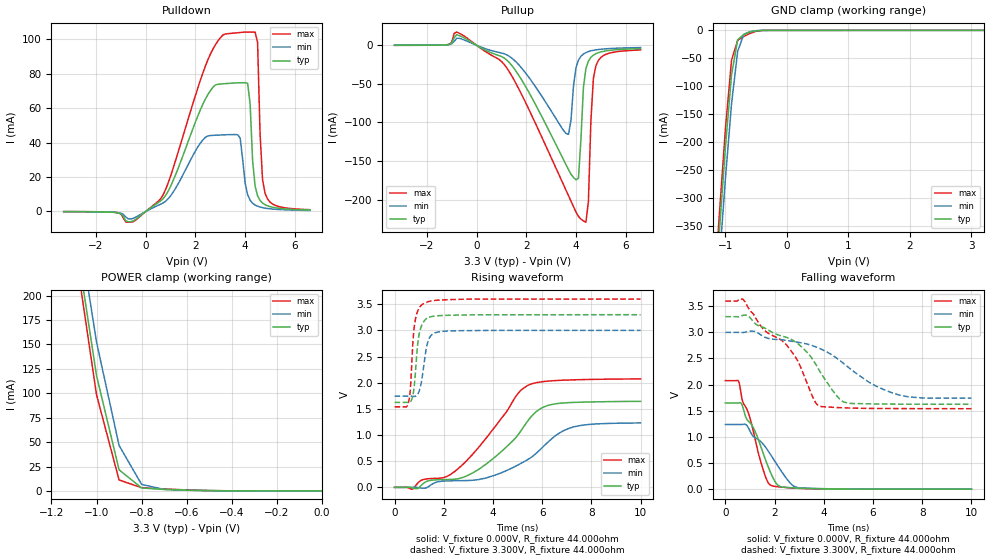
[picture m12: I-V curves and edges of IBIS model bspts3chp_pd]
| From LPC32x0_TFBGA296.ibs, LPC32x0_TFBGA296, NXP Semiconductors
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| |   Rev 0.20 IBIS Model Design Automation Generation   |
| |   N O N - S I L I C O N   C O R R E L A T E D   |
| |   This IBIS [Model] is pre-Beta tactical support   |
| |  Note: this IBIS [Model] contains clamp curves generated   |
| |   through simulation which should not be relied upon   |
| bspts3chp
|   Bidirectional Pad 3v3
|   3state Output
|   Plain Input
|   3ns Slew Rate control
|   CMOS
|   Programmable between
|   - (p1=0, p2=1) plain input
|   - (p1=0, p2=0) with Pull Up
|   - (p1=1, p2=1) with Pull Down
|   - (p1=1, p2=0) with Repeater
|   Characterized at Core 1.2V and I/O 3.3V
| Pull Down Mode (p1=1, p2=1)
[Model]   bspts3chp_pd | of bspts3chp
Model_type   I/O
Polarity   Non-Inverting
Enable   Active-Low
|  Reciever Thresholds
Vinl   = 0.36V
Vinh   = 0.84V
| AC Test Load Conditions
Vref   = 0
Cref   = 1.2e-11
Rref   = 1000000000
Vmeas   = 0.6
| [Process Range]   typical   min   max
| C_comp edge width   400.000ps   400.000ps   400.000ps
| C_comp Tstrobe   40.000fs   40.000fs   40.000fs
C_comp   2.386pF   2.237pF   2.564pF
[Temperature Range]   25   125   -40
[Voltage Range]   3.30V   3.00V   3.60V
[GND Clamp Reference]   0.00V   0.00V   0.00V
[Pulldown Reference]   0.00V   0.00V   0.00V
[POWER Clamp Reference]   3.30V   3.00V   3.60V
[Pullup Reference]   3.30V   3.00V   3.60V
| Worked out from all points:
|   slope of the pulldown table from 0 to 0.495 V, typ, clamps not added: 97.1 ohm
|   slope of the pullup table from 0 to 0.495 V, typ, clamps not added: 59.3 ohm
|   GND clamp passes 1 mA (typ) near -0.51 V on its own axis
|   POWER clamp passes 1 mA (typ) near -0.63 V on its own axis
|   rising waveform, V_fixture 0.000V, R_fixture 44.000ohm: 20-80 % time 2.13ns typ, 2.37ns min, 2.1ns max; typ from 0 V to 1.64 V
|   falling waveform, V_fixture 0.000V, R_fixture 44.000ohm: 20-80 % time 927ps typ, 1.23ns min, 792ps max; typ from 1.65 V to 0 V
|   rising waveform, V_fixture 3.300V, R_fixture 44.000ohm: 20-80 % time 212ps typ, 253ps min, 186ps max; typ from 1.62 V to 3.3 V
|   falling waveform, V_fixture 3.300V, R_fixture 44.000ohm: 20-80 % time 2.18ns typ, 2.51ns min, 2.04ns max; typ from 3.3 V to 1.62 V
[GND Clamp]
| ref voltage   0.00V   0.00V   0.00V
|   Voltage   I(typ)   I(min)   I(max)
-3.3V     -4.198A    -4.223A    -4.188A
-1.2V     -526mA     -577.5mA   -497.2mA
-1.1V     -363.6mA   -417.9mA   -332.6mA
-1V       -210.1mA   -266.3mA   -177.3mA
-900mV    -79.71mA   -131.5mA   -53.29mA
-800mV    -16.76mA   -37.38mA   -17.81mA
-700mV    -7.164mA   -7.263mA   -10.92mA
-600mV    -3.002mA   -2.202mA   -5.445mA
-500mV    -699uA     -571.9uA   -1.612mA
-400mV    -79uA      -96.04uA   -163.6uA
3.2V      50.82uA    25.42uA    83.99uA
[Power Clamp]   | Vtable = Vcc - Vpad
| ref voltage   3.30V   3.00V   3.60V
|   Voltage   I(typ)   I(min)   I(max)
-3.3V     4.52A      4.504A     4.537A
-1.1V     269.9mA    299.6mA    255.3mA
-1V       118.1mA    152.5mA    98.49mA
-900mV    21.63mA    46.53mA    11.26mA
-800mV    3.041mA    6.684mA    3.29mA
-700mV    1.546mA    1.559mA    2.017mA
-600mV    791.6uA    711.8uA    1.06mA
-400mV    91.28uA    94.64uA    124.4uA
0V        50.84uA    24.87uA    84.1uA
[Pulldown]
| ref voltage   0.00V   0.00V   0.00V
|   Voltage   I(typ)   I(min)   I(max)
-3.3V     -80.68uA   -69.9uA    -74.32uA
-600mV    -5.92mA    -4.329mA   -6.172mA
500mV     5.147mA    3.568mA    5.922mA
2.5V      67.8mA     43.83mA    87.99mA
3.7V      74.65mA    44.53mA    103.7mA
4V        74.69mA    16.44mA    104.1mA
4.2V      62.38mA    6.515mA    104mA
4.3V      29.49mA    4.769mA    104mA
4.5V      9.069mA    3.068mA    98.17mA
4.6V      6.414mA    2.587mA    45.15mA
4.8V      3.956mA    1.96mA     10.6mA
6.6V      844.9uA    597.5uA    1.056mA
[Pullup]   | Vtable = Vcc - Vpad
| ref voltage   3.30V   3.00V   3.60V
|   Voltage   I(typ)   I(min)   I(max)
-3.3V     39.4uA     37.84uA    38.83uA
-800mV    13.66mA    9.122mA    17.15mA
1V        -14.52mA   -9.936mA   -20.86mA
3.7V      -161.3mA   -115.5mA   -195.1mA
4V        -174.4mA   -29.02mA   -216.2mA
4.1V      -172.4mA   -19.17mA   -221.9mA
4.4V      -30.01mA   -9.422mA   -229.4mA
4.5V      -20.39mA   -8.135mA   -202.5mA
4.6V      -15.6mA    -7.195mA   -97.92mA
4.7V      -12.75mA   -6.48mA    -42.98mA
4.8V      -10.87mA   -5.92mA    -26.67mA
6.6V      -4.278mA   -2.929mA   -6.056mA
[Ramp]
R_load   = 44.000ohm
|   dV/dt(typ)   dV/dt(min)   dV/dt(max)
dV/dt_r   1.000V/2.135ns   750.585mV/2.380ns   1.258V/2.105ns
dV/dt_f   1.021V/2.185ns   769.127mV/2.460ns   1.253V/2.025ns
[Rising Waveform]  | cubic spline decimation from 2001 points
V_fixture   = 0.000V
R_fixture   = 44.000ohm
|   Time   V(typ)   V(min)   V(max)
0s        20.64nV    394.3nV    10.69nV
730ps     -10.48mV   1.46mV     -33.3mV
1.125ns   55.92mV    -15.1mV    142.7mV
2.46ns    156.3mV    126.8mV    308.4mV
4.095ns   583.6mV    234.4mV    1.165V
5.02ns    1.004V     428.4mV    1.795V
5.455ns   1.294V     544.2mV    1.957V
6.02ns    1.526V     768.3mV    2.02V
7.08ns    1.619V     1.126V     2.051V
10ns      1.644V     1.231V     2.072V
[Falling Waveform]  | cubic spline decimation from 2001 points
V_fixture   = 0.000V
R_fixture   = 44.000ohm
|   Time   V(typ)   V(min)   V(max)
0s        1.648V     1.237V     2.076V
535ps     1.649V     1.237V     2.063V
695ps     1.589V     1.238V     1.691V
850ps     1.357V     1.229V     1.551V
1.16ns    1.154V     998.7mV    1.057V
1.51ns    721.8mV    875.4mV    412.1mV
1.86ns    292.7mV    644.5mV    70.76mV
2.22ns    52.44mV    382.5mV    42.77mV
2.975ns   19.67mV    27.05mV    16.53mV
10ns      25.46uV    53.35uV    21.06uV
[Rising Waveform]  | cubic spline decimation from 2001 points
V_fixture   = 3.300V
V_fixture_min = 3.000V
V_fixture_max = 3.600V
R_fixture   = 44.000ohm
|   Time   V(typ)   V(min)   V(max)
0s        1.623V     1.742V     1.539V
535ps     1.623V     1.742V     1.579V
625ps     1.625V     1.742V     1.784V
700ps     1.682V     1.741V     2.362V
780ps     1.85V      1.739V     2.973V
885ps     2.429V     1.748V     3.288V
1.03ns    2.99V      1.883V     3.45V
1.32ns    3.232V     2.72V      3.539V
2.16ns    3.288V     2.988V     3.585V
10ns      3.299V     2.999V     3.598V
[Falling Waveform]  | cubic spline decimation from 2001 points
V_fixture   = 3.300V
V_fixture_min = 3.000V
V_fixture_max = 3.600V
R_fixture   = 44.000ohm
|   Time   V(typ)   V(min)   V(max)
0s        3.299V     2.999V     3.598V
735ps     3.326V     2.997V     3.624V
1.515ns   3.097V     2.929V     3.075V
2.445ns   2.908V     2.848V     2.779V
3.165ns   2.692V     2.792V     2.214V
3.825ns   2.264V     2.693V     1.589V
4.655ns   1.718V     2.459V     1.559V
5.03ns    1.642V     2.319V     1.552V
7.035ns   1.626V     1.805V     1.541V
10ns      1.624V     1.742V     1.539V
